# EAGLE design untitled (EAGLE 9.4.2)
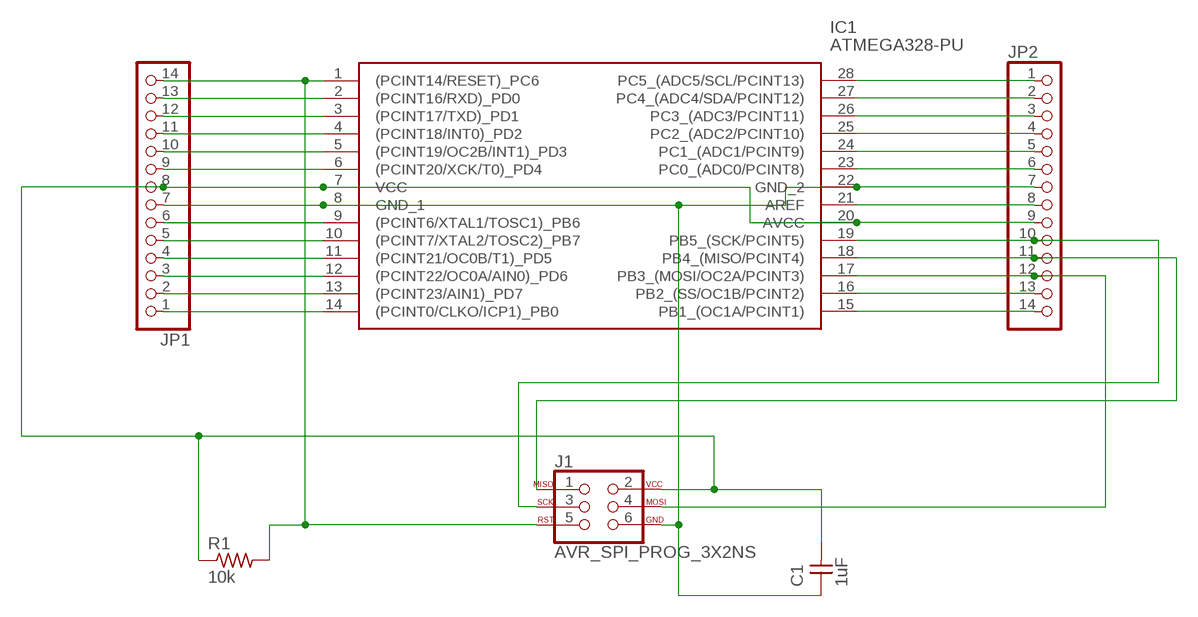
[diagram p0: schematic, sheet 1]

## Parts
C1  1uF  CAP-UNPOLARIZEDFAB  [C1206FAB]
IC1  ATMEGA328-PU  [DIP1016W53P254L3468H457Q28N]
J1  AVR_SPI_PROG_3X2NS  [2X3-NS]
JP1  PINHD-1X14  [1X14]
JP2  PINHD-1X14  [1X14]
R1  10k  RES-US1206FAB  [R1206FAB]

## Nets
N$1: IC1.28(PC5_(ADC5/SCL/PCINT13)) JP2.1
N$2: IC1.27(PC4_(ADC4/SDA/PCINT12)) JP2.2
N$3: IC1.26(PC3_(ADC3/PCINT11)) JP2.3
N$4: IC1.25(PC2_(ADC2/PCINT10)) JP2.4
N$5: IC1.24(PC1_(ADC1/PCINT9)) JP2.5
N$6: IC1.23(PC0_(ADC0/PCINT8)) JP2.6
N$8: IC1.21(AREF) JP2.8
N$10: IC1.19(PB5_(SCK/PCINT5)) J1.3 JP2.10
N$11: IC1.18(PB4_(MISO/PCINT4)) J1.1 JP2.11
N$12: IC1.17(PB3_(MOSI/OC2A/PCINT3)) J1.4 JP2.12
N$13: IC1.16(PB2_(SS/OC1B/PCINT2)) JP2.13
N$14: IC1.15(PB1_(OC1A/PCINT1)) JP2.14
N$15: IC1.14((PCINT0/CLKO/ICP1)_PB0) JP1.1
N$16: IC1.13((PCINT23/AIN1)_PD7) JP1.2
N$17: IC1.12((PCINT22/OC0A/AIN0)_PD6) JP1.3
N$18: IC1.11((PCINT21/OC0B/T1)_PD5) JP1.4
N$19: IC1.10((PCINT7/XTAL2/TOSC2)_PB7) JP1.5
N$20: IC1.9((PCINT6/XTAL1/TOSC1)_PB6) JP1.6
N$21: C1.1 IC1.8(GND_1) IC1.22(GND_2) J1.6 JP1.7 JP2.7
N$22: C1.2 IC1.7(VCC) IC1.20(AVCC) J1.2 JP1.8 JP2.9 R1.1
N$23: IC1.6((PCINT20/XCK/T0)_PD4) JP1.9
N$24: IC1.5((PCINT19/OC2B/INT1)_PD3) JP1.10
N$25: IC1.4((PCINT18/INT0)_PD2) JP1.11
N$26: IC1.3((PCINT17/TXD)_PD1) JP1.12
N$27: IC1.2((PCINT16/RXD)_PD0) JP1.13
N$28: IC1.1((PCINT14/RESET)_PC6) J1.5 JP1.14 R1.2

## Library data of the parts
C1 = fab:CAP-UNPOLARIZED
IC1 = SamacSys_Parts:ATMEGA328-PU: 8-bit Microcontrollers - MCU AVR 32K FLSH 1K EE2K SRAM-20MHz IND Source: Datasheet; DESCRIPTION: 8-bit Microcontrollers - MCU AVR 32K FLSH 1K EE2K SRAM-20MHz IND; HEIGHT: 4.572mm; MANUFACTURER_NAME: Microchip; MANUFACTURER_PART_NUMBER: ATMEGA328-PU; MOUSER_PART_NUMBER: 556-ATMEGA328-PU; MOUSER_PRICE-STOCK: https://www.mouser.com/Search/Refine.aspx?Keyword=556-ATMEGA328-PU
J1 = SparkFun-Connectors:AVR_SPI_PROG_3X2: AVR ISP 6 Pin This is the reduced ISP connector for AVR programming. Common on Arduino. This footprint will take up less PCB space and can be used with a 10-pin to 6-pin adapter such as SKU: BOB-08508 **Special note about "TEST_POINT" package. The stop mask is on the top side, so if you want your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
JP1 JP2 = pinhead+:PINHD-1X14: PIN HEADER
R1 = fab:RES-US: Resistor (US Symbol)

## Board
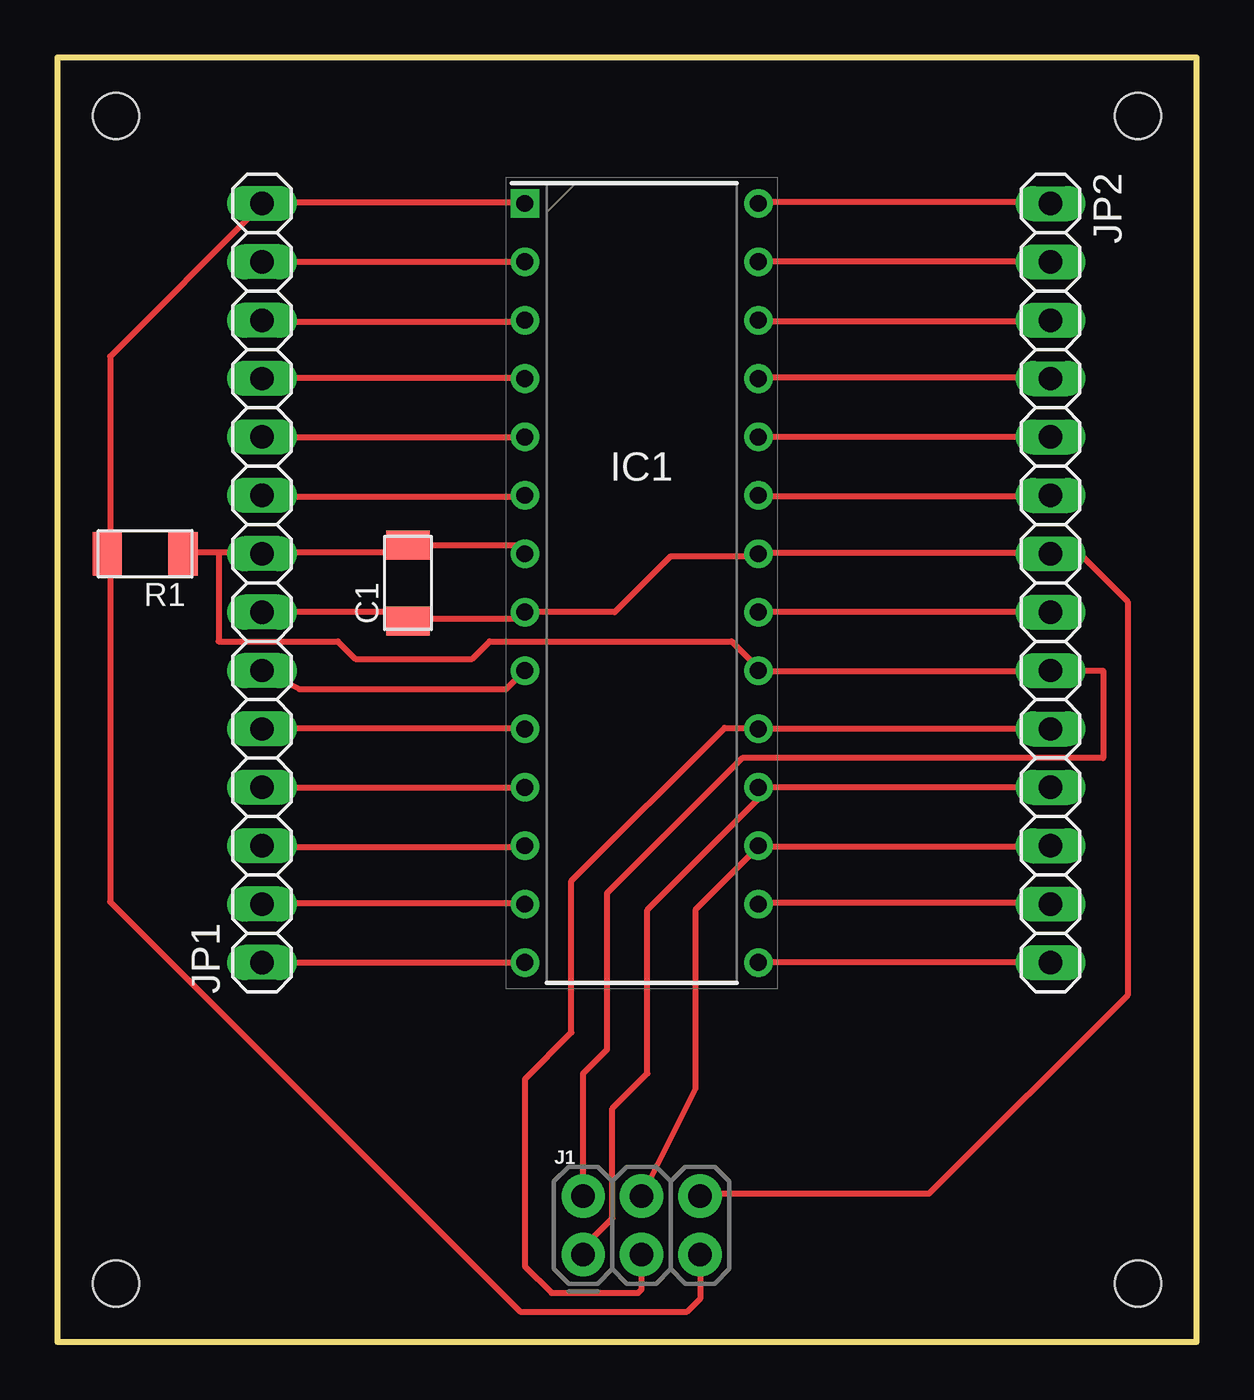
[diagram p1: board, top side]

Size 49.53 x 55.88 mm. Coordinates in mm from the lower left corner, seen from the top.
Outline: 0,55.88 49.53,55.88 49.53,0 0,0 0,55.88
Copper layers (1*16): Top 0.035mm / dielectric 1.5mm / Bottom 0.035mm
Design rules "default": minimum track width 6mil, minimum drill 0.35mm, track to track 6mil, track to pad 6mil, pad to pad 6mil, via to via 6mil, smd to smd 6mil, copper to edge 40mil, drill to drill 6mil, minimum pad ring 10mil, minimum via ring 8mil, stop-mask expansion 4mil, vias tented up to drill 0mil, thermal gap 10mil
Holes 2 mm at 2.54,53.34 46.99,53.34 46.99,2.54 2.54,2.54

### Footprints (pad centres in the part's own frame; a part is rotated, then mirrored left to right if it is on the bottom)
C1206FAB = smd 1.27 x 1.905: 1 -1.651,0; 2 1.651,0
DIP1016W53P254L3468H457Q28N = drill 0.733 pad 1.133 square: 1 -5.08,16.51 | drill 0.733 pad 1.133: 2 -5.08,13.97; 3 -5.08,11.43; 4 -5.08,8.89; 5 -5.08,6.35; 6 -5.08,3.81; 7 -5.08,1.27; 8 -5.08,-1.27; 9 -5.08,-3.81; 10 -5.08,-6.35; 11 -5.08,-8.89; 12 -5.08,-11.43; 13 -5.08,-13.97; 14 -5.08,-16.51; 15 5.08,-16.51; 16 5.08,-13.97; 17 5.08,-11.43; 18 5.08,-8.89; 19 5.08,-6.35; 20 5.08,-3.81; 21 5.08,-1.27; 22 5.08,1.27; 23 5.08,3.81; 24 5.08,6.35; 25 5.08,8.89; 26 5.08,11.43; 27 5.08,13.97; 28 5.08,16.51
2X3-NS = drill 1.016 pad 1.88: 1 -2.54,-1.27; 2 -2.54,1.27; 3 0,-1.27; 4 0,1.27; 5 2.54,-1.27; 6 2.54,1.27
1X14 = drill 1.016 long: 1 -16.51,0; 2 -13.97,0; 3 -11.43,0; 4 -8.89,0; 5 -6.35,0; 6 -3.81,0; 7 -1.27,0; 8 1.27,0; 9 3.81,0; 10 6.35,0; 11 8.89,0; 12 11.43,0; 13 13.97,0; 14 16.51,0
R1206FAB = smd 1.27 x 1.905: 1 -1.651,0; 2 1.651,0

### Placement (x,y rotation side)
C1  15.24,33.02 90 top
IC1  25.4,33.02 0 top
J1  25.4,5.08 0 top
JP1  8.89,33.02 90 top
JP2  43.18,33.02 270 top
R1  3.81,34.29 180 top

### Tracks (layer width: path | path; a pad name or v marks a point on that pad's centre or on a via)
N$1
  Top 0.254: IC1.28 30.48,49.58 43.13,49.58 JP2.1
N$2
  Top 0.254: JP2.2 IC1.27
N$3
  Top 0.254: IC1.26 30.48,44.4 43.13,44.4 JP2.3
N$4
  Top 0.254: IC1.25 30.48,41.96 43.13,41.96 JP2.4
N$5
  Top 0.254: JP2.5 IC1.24
N$6
  Top 0.254: IC1.23 30.48,36.78 43.13,36.78 JP2.6
N$8
  Top 0.254: JP2.8 IC1.21
N$10
  Top 0.254: J1.3 25.4,2.29 25.25,2.13 21.49,2.13 20.32,3.3 20.32,11.43 22.35,13.46 22.35,20.07 29.01,26.72 30.43,26.72 IC1.19 JP2.10
N$11
  Top 0.254: JP2.11 IC1.18 30.48,23.62 25.65,18.8 25.65,11.68 24.13,10.16 24.13,5.38 22.86,4.12 J1.1
N$12
  Top 0.254: 30.48,21.54 43.13,21.54 JP2.12 | 30.48,21.54 27.74,18.8 27.74,11.02 J1.4 | 30.48,21.54 IC1.17
N$13
  Top 0.254: IC1.16 30.48,19.1 43.13,19.1 JP2.13
N$14
  Top 0.254: JP2.14 IC1.15
N$15
  Top 0.254: JP1.1 IC1.14
N$16
  Top 0.254: IC1.13 20.27,19.1 8.99,19.1 JP1.2
N$17
  Top 0.254: IC1.12 20.27,21.54 8.99,21.54 JP1.3
N$18
  Top 0.254: JP1.4 IC1.11
N$19
  Top 0.254: IC1.10 20.27,26.72 8.99,26.72 JP1.5
N$20
  Top 0.254: IC1.9 19.51,28.4 10.52,28.4 JP1.6
N$21
  Top 0.254: 15.24,31.45 19.96,31.45 20.27,31.75 IC1.8 24.23,31.75 26.67,34.19 30.48,34.19 IC1.22 30.48,34.34 43.13,34.34 JP2.7 44.45,34.29 46.53,32.21 46.53,15.09 37.9,6.45 28.04,6.45 J1.6 | JP1.7 14.94,31.75 15.24,31.45 | 15.24,31.45 C1.1
N$22
  Top 0.254: 7.01,34.34 8.84,34.34 JP1.8 8.99,34.34 14.94,34.34 15.24,34.65 | 7.01,34.34 5.49,34.34 R1.1 | 15.24,34.65 19.96,34.65 IC1.7 | 15.24,34.65 C1.2 | 7.01,34.34 7.01,30.48 12.19,30.48 12.95,29.72 18.03,29.72 18.8,30.48 29.31,30.48 30.48,29.31 IC1.20 30.48,29.16 43.13,29.16 JP2.9 45.47,29.21 45.47,25.4 29.77,25.4 23.9,19.53 23.9,12.73 22.86,11.68 J1.2
N$23
  Top 0.254: IC1.6 20.27,36.78 8.99,36.78 JP1.9
N$24
  Top 0.254: JP1.10 IC1.5
N$25
  Top 0.254: IC1.4 20.27,41.96 8.99,41.96 JP1.11
N$26
  Top 0.254: IC1.3 20.27,44.4 8.99,44.4 JP1.12
N$27
  Top 0.254: JP1.13 IC1.2
N$28
  Top 0.254: IC1.1 20.27,49.58 8.99,49.58 JP1.14 8.84,49.43 2.29,42.88 2.29,34.34 R1.2 2.29,34.19 2.29,19.15 20.12,1.32 27.38,1.32 27.94,1.88 J1.5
